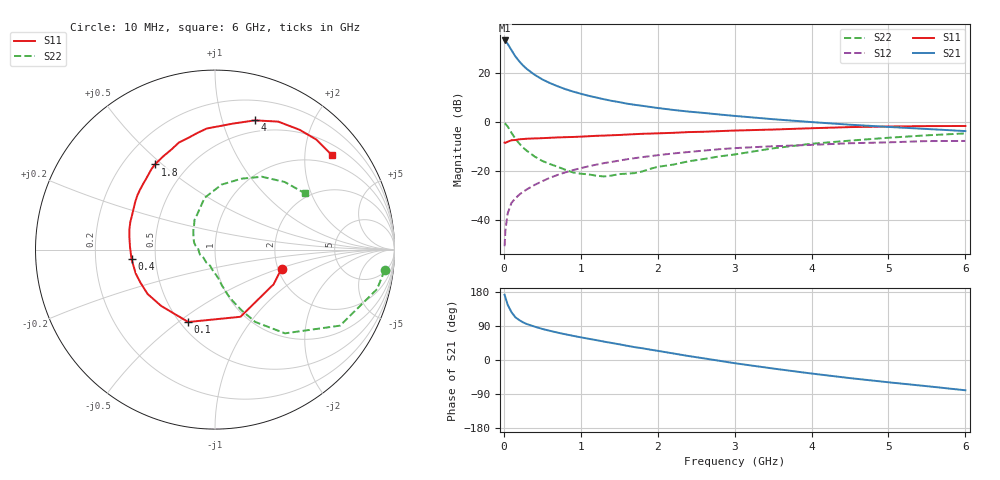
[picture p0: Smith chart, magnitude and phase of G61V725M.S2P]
! SIEMENS Small Signal Semiconductors
! BFG193
! Si NPN RF Bipolar Junction Transistor in SOT223
! VCE = 1.75 V  IC = 25 mA
! Common Emitter S-Parameters:  August  1996
# GHz  S  MA  R  50
!  f  S11  S21  S12  S22
! GHz  MAG  ANG  MAG  ANG  MAG  ANG  MAG  ANG
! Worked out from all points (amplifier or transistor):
!   36 points, 10 MHz to 6 GHz, reference 50 ohm
!   highest |S21| = 33.3 dB at 10 MHz (marker M1)
!   |S21| within 3 dB of that: start of sweep to 81.07 MHz
!   unconditionally stable (mu >= 1): 580.7 MHz to 2.67 GHz
!   at 250 MHz: K = 0.81, MSG = 25.7 dB, |S12| = -28.3 dB
!   at 1.4 GHz: K = 1.05, MAG = 11.0 dB, |S12| = -16.2 dB
!   at 6 GHz: K = 0.93, MSG = 2.0 dB, |S12| = -7.6 dB
!   S11 on the Smith chart (normalised r, x): 10 MHz: 2.09, -0.52; 100 MHz: 0.55, -0.54; 400 MHz: 0.36, -0.05; 1.8 GHz: 0.33, +0.47; 4 GHz: 0.38, +1.28; 6 GHz: 0.75, +2.64
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0.01  0.3855 -16.0  46.11 172.1  0.003 85.8  0.9526 -6.9
0.02  0.3795 -30.6  44.98 165.4  0.0062 81.3  0.9293 -13.7
0.05  0.4003 -69.2  39.32 145.7  0.014 68.7  0.8155 -31.3
0.1  0.43 -110.3  29.15 125.9  0.0229 61.9  0.6081 -50.1
0.15  0.434 -133.6  21.82 112.8  0.0282 57.7  0.4613 -60.9
0.2  0.4496 -146.6  17.38 105.3  0.0335 58.4  0.3699 -66.3
0.25  0.4543 -156.0  14.23 99.3  0.0383 59.3  0.303 -71.0
0.3  0.4613 -163.1  12.08 94.8  0.0431 60.6  0.2615 -74.2
0.4  0.4678 -173.4  9.243 88.1  0.053 61.5  0.2002 -79.4
0.5  0.4737 178.4  7.432 82.0  0.063 61.2  0.1627 -83.1
0.6  0.4816 171.9  6.251 77.0  0.0743 60.8  0.1406 -87.7
0.7  0.4903 166.7  5.387 72.2  0.0846 60.4  0.1237 -93.7
0.9  0.5008 157.1  4.203 63.7  0.106 57.3  0.0948 -106.1
1.1  0.5179 149.1  3.457 56.1  0.1265 54.3  0.0869 -123.7
1.4  0.5424 137.6  2.726 45.0  0.1556 48.1  0.0821 -153.9
1.8  0.5807 125.2  2.156 31.0  0.1947 39.7  0.0996 173.2
2.2  0.6079 113.6  1.78 17.4  0.2312 30.4  0.137 151.2
3.5  0.7091 81.9  1.151 -22.5  0.3246 -1.0  0.2942 101.4
4  0.7538 72.8  1.006 -35.7  0.3457 -10.7  0.3642 84.2
4.5  0.7954 63.7  0.889 -47.8  0.3733 -20.6  0.4219 69.5
5.5  0.8337 47.2  0.728 -69.1  0.4129 -43.5  0.5412 44.1
6  0.8376 38.9  0.66 -79.9  0.4158 -56.5  0.592 31.9
